| IBIS file stm32wl33_vfqfpn48.ibs
[IBIS ver] 4.2
[File name] stm32wl33_vfqfpn48.ibs
[File Rev] 1.0
[Date]  24-06-2024
[Source] Data Created at STMicroelectronics
[Notes]  File originated from ELDO simulations.
[Disclaimer]  This information is for modeling purpose only and is
   not guaranteed. The information is subject to change without
   notice.
[Copyright] Copyright 2024 STMicroelectronics Inc.
|   Component stm32wl33_vfqfpn48
[Component] stm32wl33_vfqfpn48
[Manufacturer] STMicroelectronics
[Package]
| variable   typ   min   max
R_pkg  0  NA  NA
L_pkg  0  NA  NA
C_pkg  0  NA  NA
[Pin]   signal_name   model_name
1  PA2  io8prog2m25m50m120m_sudq_ft
2  PA3  io8prog2m25m50m120m_sudq_ft
3  VDD_1  power
4  PB3  io8prog2m25m50m120m_sudq_ft
5  PB4  io8prog2m25m50m120m_sudq_ft
6  PB5  io8prog2m25m50m120m_sudq_ft
7  PA0  io8prog2m25m50m120m_sudq_i2c_ft
8  PA4  io8prog2m25m50m120m_sudq_ft
9  PA11  io8prog2m25m50m120m_sudq_ft
10  PA10  io8prog2m25m50m120m_sudq_ft
11  PA9  io8prog2m25m50m120m_sudq_ft
12  PA8  io8prog2m25m50m120m_sudq_ft
13  PB6  io8prog2m25m50m120m_sudq_i2c_ft
14  PA5  io8prog2m25m50m120m_sudq_ft
15  PA6  io8prog2m25m50m120m_sudq_i2c_ft
16  PA7  io8prog2m25m50m120m_sudq_i2c_ft
17  PB12  io8prog2m25m50m120m_sudq_ft
18  PB13  io8prog2m25m50m120m_sudq_ft
19  PB14  io8prog2m25m50m120m_sudq_ft
20  PB15  io8prog2m25m50m120m_sudq_ft
21  VDD_2  power
22  LPAWUR  nc
23  RX  nc
24  EXTGND  gnd
25  TX_HP  nc
26  TX  nc
27  VDDRF  nc
28  OSCOUT  nc
29  OSCIN  nc
30  PA1  io8prog2m25m50m120m_sudq_i2c_ft
31  PB7  io8prog2m25m50m120m_sudq_i2c_ft
32  PB11  io8prog2m25m50m120m_sudq_i2c_ft
33  PB10  io8prog2m25m50m120m_sudq_i2c_ft
34  PB9  io8prog2m25m50m120m_sudq_ft
35  PB8  io8prog2m25m50m120m_sudq_ft
36  NRST  nc
37  VDDSD  nc
38  VLXSD  nc
39  VSSSD  nc
40  VFBSD  nc
41  VCAP  nc
42  PA12  io8prog2m25m50m120m_sudq_ft
43  PA13  io8prog2m25m50m120m_sudq_i2c_ft
44  PA14  io8prog2m25m50m120m_sudq_i2c_ft
45  PA15  io8prog2m25m50m120m_sudq_ft
46  PB0  io8prog2m25m50m120m_sudq_ft
47  PB1  io8prog2m25m50m120m_sudq_ft
48  PB2  io8prog2m25m50m120m_sudq_ft
0  EXTGND  gnd
[Package Model]   4l0-qfn-6x6-48-100mhz-230713
[Pin Mapping]   pulldown_ref   pullup_ref   | Comment
1  gndio  vddio
2  gndio  vddio
3  nc  vddio
4  gndio  vddio
5  gndio  vddio
6  gndio  vddio
7  gndio  vddio
8  gndio  vddio
9  gndio  vddio
10  gndio  vddio
11  gndio  vddio
12  gndio  vddio
13  gndio  vddio
14  gndio  vddio
15  gndio  vddio
16  gndio  vddio
17  gndio  vddio
18  gndio  vddio
19  gndio  vddio
20  gndio  vddio
21  nc  vddio
22  nc  nc
23  nc  nc
24  gndio  nc
25  nc  nc
26  nc  nc
27  nc  nc
28  nc  nc
29  nc  nc
30  gndio  vddio
31  gndio  vddio
32  gndio  vddio
33  gndio  vddio
34  gndio  vddio
35  gndio  vddio
36  nc  nc
37  nc  nc
38  nc  nc
39  nc  nc
40  nc  nc
41  nc  nc
42  gndio  vddio
43  gndio  vddio
44  gndio  vddio
45  gndio  vddio
46  gndio  vddio
47  gndio  vddio
48  gndio  vddio
0  gndio  nc
[Model Selector] io8prog2m25m50m120m_sudq_ft
iols8p_sudq_ft_pd_lv  "IO low speed, PD=40kOhm - 1P8V"
iols8p_sudq_ft_pu_lv  "IO low speed, PU=40kOhm - 1P8V"
iols8p_sudq_ft_lv  "IO low speed - 1P8V"
iols8p_sudq_ft_pd  "IO low speed, PD=40kOhm - 3P3V"
iols8p_sudq_ft_pu  "IO low speed, PU=40kOhm - 3P3V"
iols8p_sudq_ft  "IO low speed - 3P3V"
iofs8p_sudq_ft_pd_lv  "IO full speed, PD=40kOhm - 1P8V"
iofs8p_sudq_ft_pu_lv  "IO full speed, PU=40kOhm - 1P8V"
iofs8p_sudq_ft_lv  "IO full speed - 1P8V"
iofs8p_sudq_ft_pd  "IO full speed, PD=40kOhm - 3P3V"
iofs8p_sudq_ft_pu  "IO full speed, PU=40kOhm - 3P3V"
iofs8p_sudq_ft  "IO full speed - 3P3V"
ioms8p_sudq_ft_pd_lv  "IO medium speed, PD=40kOhm - 1P8V"
ioms8p_sudq_ft_pu_lv  "IO medium speed, PU=40kOhm - 1P8V"
ioms8p_sudq_ft_lv  "IO medium speed - 1P8V"
ioms8p_sudq_ft_pd  "IO medium speed, PD=40kOhm - 3P3V"
ioms8p_sudq_ft_pu  "IO medium speed, PU=40kOhm - 3P3V"
ioms8p_sudq_ft  "IO medium speed - 3P3V"
iohs8p_sudq_ft_pd_lv  "IO high speed, PD=40kOhm - 1P8V"
iohs8p_sudq_ft_pu_lv  "IO high speed, PU=40kOhm - 1P8V"
iohs8p_sudq_ft_lv  "IO high speed - 1P8V"
iohs8p_sudq_ft_pd  "IO high speed, PD=40kOhm - 3P3V"
iohs8p_sudq_ft_pu  "IO high speed, PU=40kOhm - 3P3V"
iohs8p_sudq_ft  "IO high speed - 3P3V"
[Model Selector] io8prog2m25m50m120m_sudq_i2c_ft
iols8p_sudq_ft_pd_lv  "IO low speed, PD=40kOhm - 1P8V"
iols8p_sudq_ft_pu_lv  "IO low speed, PU=40kOhm - 1P8V"
iols8p_sudq_ft_lv  "IO low speed - 1P8V"
iols8p_sudq_ft_pd  "IO low speed, PD=40kOhm - 3P3V"
iols8p_sudq_ft_pu  "IO low speed, PU=40kOhm - 3P3V"
iols8p_sudq_ft  "IO low speed - 3P3V"
iofs8p_sudq_ft_pd_lv  "IO full speed, PD=40kOhm - 1P8V"
iofs8p_sudq_ft_pu_lv  "IO full speed, PU=40kOhm - 1P8V"
iofs8p_sudq_ft_lv  "IO full speed - 1P8V"
iofs8p_sudq_ft_pd  "IO full speed, PD=40kOhm - 3P3V"
iofs8p_sudq_ft_pu  "IO full speed, PU=40kOhm - 3P3V"
iofs8p_sudq_ft  "IO full speed - 3P3V"
ioms8p_sudq_ft_pd_lv  "IO medium speed, PD=40kOhm - 1P8V"
ioms8p_sudq_ft_pu_lv  "IO medium speed, PU=40kOhm - 1P8V"
ioms8p_sudq_ft_lv  "IO medium speed - 1P8V"
ioms8p_sudq_ft_pd  "IO medium speed, PD=40kOhm - 3P3V"
ioms8p_sudq_ft_pu  "IO medium speed, PU=40kOhm - 3P3V"
ioms8p_sudq_ft  "IO medium speed - 3P3V"
iohs8p_sudq_ft_pd_lv  "IO high speed, PD=40kOhm - 1P8V"
iohs8p_sudq_ft_pu_lv  "IO high speed, PU=40kOhm - 1P8V"
iohs8p_sudq_ft_lv  "IO high speed - 1P8V"
iohs8p_sudq_ft_pd  "IO high speed, PD=40kOhm - 3P3V"
iohs8p_sudq_ft_pu  "IO high speed, PU=40kOhm - 3P3V"
iohs8p_sudq_ft  "IO high speed - 3P3V"
io8_ft_i2c_ls_1v2   "GPIO I2C open-drain - 5V tolerant - 1.2V range - Low speed"
io8_ft_i2c_ms_1v2   "GPIO I2C open-drain - 5V tolerant - 1.2V range - Med speed"
io8_ft_i2c_fs_1v2   "GPIO I2C open-drain - 5V tolerant - 1.2V range - Fast speed"
io8_ft_i2c_hs_1v2   "GPIO I2C open-drain - 5V tolerant - 1.2V range - High speed"
io8_ft_i2c_ls_1v8   "GPIO I2C open-drain - 5V tolerant - 1.8V range - Low speed"
io8_ft_i2c_ms_1v8   "GPIO I2C open-drain - 5V tolerant - 1.8V range - Med speed"
io8_ft_i2c_fs_1v8   "GPIO I2C open-drain - 5V tolerant - 1.8V range - Fast speed"
io8_ft_i2c_hs_1v8   "GPIO I2C open-drain - 5V tolerant - 1.8V range - High speed"
io8_ft_i2c_ls_3v3   "GPIO I2C open-drain - 5V tolerant - 3.3V range - Low speed"
io8_ft_i2c_ms_3v3   "GPIO I2C open-drain - 5V tolerant - 3.3V range - Med speed"
io8_ft_i2c_fs_3v3   "GPIO I2C open-drain - 5V tolerant - 3.3V range - Fast speed"
io8_ft_i2c_hs_3v3   "GPIO I2C open-drain - 5V tolerant - 3.3V range - High speed"
io8_ft_i2c_fmp_3v3   "GPIO I2C open-drain fm+ - 5V tolerant - 3.3V range"
[Define Package Model]  4l0-qfn-6x6-48-100mhz-230713
[Manufacturer]  Unknown
[OEM]  Unknown
[Description]  None
[Number Of Pins]  48
[Pin Numbers]
| Pin Num   Terminal Name
22 | LPAWUR
7 | PA0
30 | PA1
1 | PA2
2 | PA3
8 | PA4
14 | PA5
15 | PA6
16 | PA7
12 | PA8
11 | PA9
10 | PA10
9 | PA11
42 | PA12
43 | PA13
44 | PA14
45 | PA15
46 | PB0
47 | PB1
48 | PB2
4 | PB3
5 | PB4
6 | PB5
13 | PB6
31 | PB7
35 | PB8
34 | PB9
33 | PB10
32 | PB11
17 | PB12
18 | PB13
19 | PB14
20 | PB15
29 | OSCIN
28 | OSCOUT
39 | VSSSD
36 | NRST
23 | RX
40 | VFBSD
38 | VLXSD
26 | TX
25 | TX_HP
27 | VDDRF
21 | VDD_2
3 | VDD_1
41 | VCAP
37 | VDDSD
24 | EXTGND
[Model Data]
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[End Model Data]
[End Package Model]
| Models and submodels in the file (37): iols8p_sudq_ft_pd_lv (I/O), iols8p_sudq_ft_pu_lv (I/O), iols8p_sudq_ft_lv (I/O), iols8p_sudq_ft_pd (I/O), iols8p_sudq_ft_pu (I/O), iols8p_sudq_ft (I/O), iofs8p_sudq_ft_pd_lv (I/O), iofs8p_sudq_ft_pu_lv (I/O), iofs8p_sudq_ft_lv (I/O), iofs8p_sudq_ft_pd (I/O), iofs8p_sudq_ft_pu (I/O), iofs8p_sudq_ft (I/O), ioms8p_sudq_ft_pd_lv (I/O), ioms8p_sudq_ft_pu_lv (I/O), ioms8p_sudq_ft_lv (I/O), ioms8p_sudq_ft_pd (I/O), ioms8p_sudq_ft_pu (I/O), ioms8p_sudq_ft (I/O), iohs8p_sudq_ft_pd_lv (I/O), iohs8p_sudq_ft_pu_lv (I/O), iohs8p_sudq_ft_lv (I/O), iohs8p_sudq_ft_pd (I/O), iohs8p_sudq_ft_pu (I/O), iohs8p_sudq_ft (I/O), io8_ft_i2c_fs_1v2 (I/O_open_drain), io8_ft_i2c_hs_1v2 (I/O_open_drain), io8_ft_i2c_ls_1v2 (I/O_open_drain), io8_ft_i2c_ms_1v2 (I/O_open_drain), io8_ft_i2c_fs_1v8 (I/O_open_drain), io8_ft_i2c_hs_1v8 (I/O_open_drain), io8_ft_i2c_ls_1v8 (I/O_open_drain), io8_ft_i2c_ms_1v8 (I/O_open_drain), io8_ft_i2c_fs_3v3 (I/O_open_drain), io8_ft_i2c_hs_3v3 (I/O_open_drain), io8_ft_i2c_ls_3v3 (I/O_open_drain), io8_ft_i2c_ms_3v3 (I/O_open_drain), io8_ft_i2c_fmp_3v3 (I/O_open_drain)
